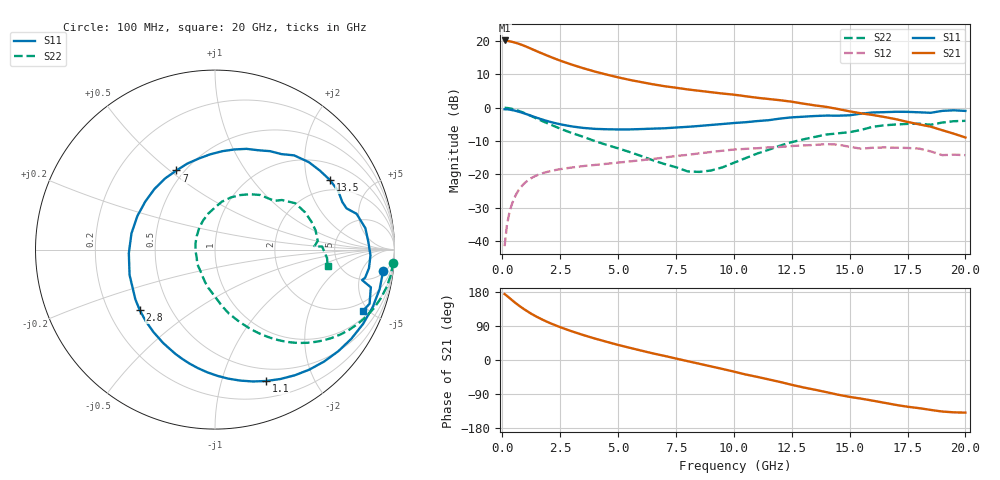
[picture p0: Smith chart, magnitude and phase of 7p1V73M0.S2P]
! Infineon Technologies  Discrete & RF Semiconductors
! bfp620
! VCE =  1.7 V,  IC =  3.0 mA
! Common Emitter S-Parameters:  Sep 2002
# GHz  S  MA  R  50
!  f  S11  S21  S12  S22
! GHz  MAG  ANG  MAG  ANG  MAG  ANG  MAG  ANG
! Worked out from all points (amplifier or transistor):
!   59 points, 100 MHz to 20 GHz, reference 50 ohm
!   highest |S21| = 20.1 dB at 100 MHz (marker M1)
!   |S21| within 3 dB of that: start of sweep to 1.415 GHz
!   unconditionally stable (mu >= 1): 5.379 GHz to 12.33 GHz; 14.32 GHz to 15.59 GHz; 17.33 GHz to end of sweep
!   at 1 GHz: K = 0.21, MSG = 20.4 dB, |S12| = -22.4 dB
!   at 5.5 GHz: K = 1.01, MAG = 11.5 dB, |S12| = -16.1 dB
!   at 20 GHz: K = 1.39, MAG = -1.1 dB, |S12| = -14.2 dB
!   S11 on the Smith chart (normalised r, x): 100 MHz: 6, -13; 1.1 GHz: 0.37, -1.40; 2.8 GHz: 0.33, -0.32; 7 GHz: 0.45, +0.53; 13.5 GHz: 1.58, +2.78; 20 GHz: 1.38, -4.63
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0.1  0.9446 -7.1  10.15 174.1  0.0084 84.3  0.9958 -4.2
0.3  0.9353 -20.1  9.88 164.1  0.0261 79.3  0.9785 -12.4
0.5  0.9076 -33.2  9.523 153.9  0.0427 71.9  0.9433 -20.3
0.6  0.8902 -39.5  9.312 149.1  0.0504 68.3  0.9211 -24.0
0.8  0.8507 -51.8  8.829 140.0  0.0642 61.5  0.8708 -30.9
1.1  0.7859 -68.7  8.017 127.8  0.081 52.4  0.7883 -39.9
1.5  0.7035 -88.9  6.978 113.7  0.0971 42.8  0.6824 -49.5
1.9  0.6356 -106.7  6.108 101.8  0.108 35.6  0.5923 -56.9
2.4  0.5733 -126.7  5.214 89.0  0.118 28.8  0.5012 -64.4
2.8  0.5382 -141.1  4.661 80.1  0.1239 24.5  0.4418 -69.6
3.5  0.4965 -163.5  3.893 65.8  0.1332 18.3  0.3654 -77.7
4  0.4805 -177.6  3.467 56.6  0.1384 14.6  0.3153 -83.1
5  0.4712 156.6  2.844 39.8  0.15 9.0  0.2456 -93.0
6  0.4775 134.8  2.412 24.8  0.163 3.6  0.1883 -107.3
7  0.4904 116.0  2.096 10.9  0.1785 -1.6  0.1431 -125.0
8.5  0.5312 93.0  1.789 -9.8  0.2062 -11.5  0.1089 -175.6
10.5  0.604 66.4  1.482 -38.1  0.241 -29.3  0.1747 112.6
12  0.6855 50.0  1.291 -58.0  0.2574 -41.8  0.27 81.8
13.5  0.7488 31.1  1.081 -78.4  0.2764 -56.5  0.3643 57.9
15  0.768 17.4  0.88 -97.3  0.2587 -76.0  0.4289 39.3
17  0.8668 -2.1  0.671 -118.5  0.2507 -87.4  0.5588 16.3
20  0.8926 -22.5  0.357 -138.9  0.1941 -105.1  0.634 -8.3
